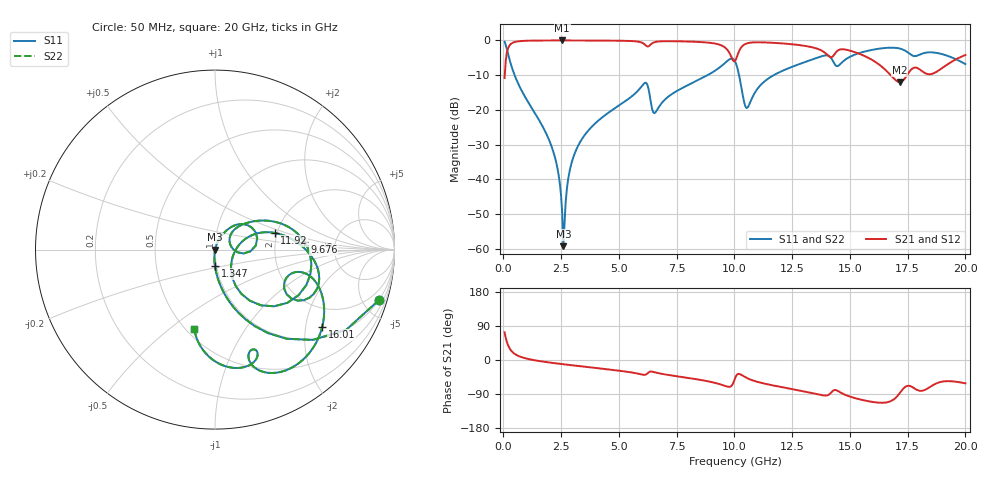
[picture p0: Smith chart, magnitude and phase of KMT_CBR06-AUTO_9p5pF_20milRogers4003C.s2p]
! Data measured by Modelithics Inc. support@modelithics.com 813-866-6335
! KEMET CBR06-AUTO 9.5pF, Pad Width= 0.851mm, Pad Length= 0.64mm, Pad Gap= 0.62mm, 20mil Rogers 4003C substrate Data, January 2022
# hz S ma R 50
! 2 Port Network Data from SP1.SP block
! freq  magS11  angS11  magS21  angS21  magS12  angS12  magS22  angS22
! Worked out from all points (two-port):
!   401 points, 50 MHz to 20 GHz, reference 50 ohm
!   highest |S21| = -0.01 dB at 2.544 GHz (marker M1); lowest = -12.0 dB at 17.16 GHz (marker M2)
!   |S21| within 3 dB of the highest: 169.2 MHz to 9.728 GHz (9.559 GHz wide, 193 % of centre); 10.21 GHz to 13.8 GHz (3.588 GHz wide, 29.9 % of centre)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
!   lowest |S11| = -59.3 dB at 2.594 GHz (marker M3), VSWR 1.00, Z = 50.1 - j0.0694 ohm
!   |S11| at or under -10 dB: 483 MHz to 8.84 GHz (8.357 GHz wide, 179 % of centre); 10.2 GHz to 11.7 GHz (1.506 GHz wide, 13.8 % of centre)
!   |S22| runs from -59.3 to -0.4 dB; largest |S21 - S12| = 0
!   S11 on the Smith chart (normalised r, x): 50 MHz: 0.98, -6.57; 1.347 GHz: 0.98, -0.18; 9.676 GHz: 2.96, +0.34; 11.92 GHz: 1.94, +0.41; 16.01 GHz: 1.32, -2.48; 20 GHz: 0.55, -0.61
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5e7  0.9576 -16.9  0.2879 73.0  0.2879 73.0  0.9576 -16.9
4.49e8  0.3386 -72.1  0.9403 17.8  0.9403 17.8  0.3386 -72.1
1.34675e9  0.09136 -90.2  0.995 -0.6  0.995 -0.6  0.09136 -90.2
2.194625e9  0.02281 -96.0  0.9988 -8.2  0.9988 -8.2  0.02281 -96.0
2.394125e9  0.01127 -95.1  0.9989 -9.8  0.9989 -9.8  0.01127 -95.1
2.54375e9  0.003271 -84.0  0.999 -10.9  0.999 -10.9  0.003271 -84.0
2.593625e9  0.001089 -39.5  0.9989 -11.2  0.9989 -11.2  0.001089 -39.5
2.94275e9  0.01688 72.8  0.9987 -13.7  0.9987 -13.7  0.01688 72.8
3.391625e9  0.03768 71.4  0.998 -16.9  0.998 -16.9  0.03768 71.4
6.084875e9  0.2389 30.8  0.8924 -39.2  0.8924 -39.2  0.2389 30.8
6.483875e9  0.09231 9.6  0.9283 -31.3  0.9283 -31.3  0.09231 9.6
6.73325e9  0.1104 40.9  0.9673 -35.1  0.9673 -35.1  0.1104 40.9
9.675875e9  0.5004 4.9  0.7446 -69.9  0.7446 -69.9  0.5004 4.9
1.0025e10  0.5007 -36.3  0.5048 -48.6  0.5048 -48.6  0.5007 -36.3
1.052375e10  0.1062 -21.1  0.9031 -47.1  0.9031 -47.1  0.1062 -21.1
1.192025e10  0.3446 15.7  0.9132 -70.1  0.9132 -70.1  0.3446 15.7
1.336662e10  0.5313 -3.1  0.7969 -87.5  0.7969 -87.5  0.5313 -3.1
1.4414e10  0.4281 -25.9  0.6857 -79.8  0.6857 -79.8  0.4281 -25.9
1.601e10  0.7365 -35.8  0.5127 -110.9  0.5127 -110.9  0.7365 -35.8
1.670825e10  0.7854 -51.7  0.3308 -110.0  0.3308 -110.0  0.7854 -51.7
1.715712e10  0.7642 -64.0  0.251 -87.4  0.251 -87.4  0.7642 -64.0
2e10  0.4563 -104.7  0.6164 -61.5  0.6164 -61.5  0.4563 -104.7
